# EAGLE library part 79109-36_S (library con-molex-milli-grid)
RECEPTACAL
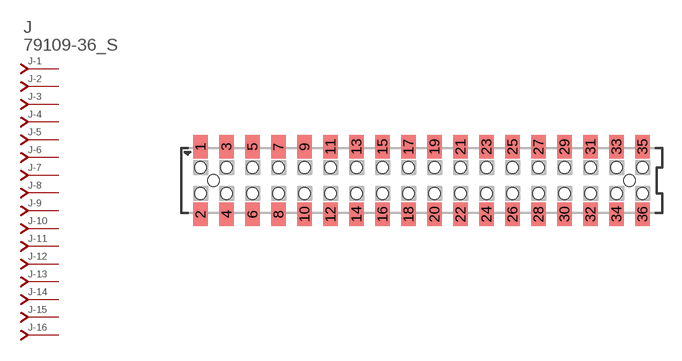
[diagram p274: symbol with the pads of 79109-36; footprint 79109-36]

Designator prefix J; gates -1=J-NV -2=J-N -3=J-N -4=J-N -5=J-N -6=J-N -7=J-N -8=J-N -9=J-N -10=J-N -11=J-N -12=J-N -13=J-N -14=J-N -15=J-N -16=J-N -17=J-N -18=J-N -19=J-N -20=J-N -21=J-N -22=J-N -23=J-N -24=J-N -25=J-N -26=J-N -27=J-N -28=J-N -29=J-N -30=J-N -31=J-N -32=J-N -33=J-N -34=J-N -35=J-N -36=J-N

## 79109-36_S  [79109-36]
1  -1:J  pas
2  -2:J  pas
3  -3:J  pas
4  -4:J  pas
5  -5:J  pas
6  -6:J  pas
7  -7:J  pas
8  -8:J  pas
9  -9:J  pas
10  -10:J  pas
11  -11:J  pas
12  -12:J  pas
13  -13:J  pas
14  -14:J  pas
15  -15:J  pas
16  -16:J  pas
17  -17:J  pas
18  -18:J  pas
19  -19:J  pas
20  -20:J  pas
21  -21:J  pas
22  -22:J  pas
23  -23:J  pas
24  -24:J  pas
25  -25:J  pas
26  -26:J  pas
27  -27:J  pas
28  -28:J  pas
29  -29:J  pas
30  -30:J  pas
31  -31:J  pas
32  -32:J  pas
33  -33:J  pas
34  -34:J  pas
35  -35:J  pas
36  -36:J  pas

## Footprint 79109-36 (pad centres in mm)
RECEPTACAL SMD Dual Row, Vertical, Pass-Thru
smd 1.12 x 1.83: 1 -17,2.6; 2 -17,-2.6; 3 -15,2.6; 4 -15,-2.6; 5 -13,2.6; 6 -13,-2.6; 7 -11,2.6; 8 -11,-2.6; 9 -9,2.6; 10 -9,-2.6; 11 -7,2.6; 12 -7,-2.6; 13 -5,2.6; 14 -5,-2.6; 15 -3,2.6; 16 -3,-2.6; 17 -1,2.6; 18 -1,-2.6; 19 1,2.6; 20 1,-2.6; 21 3,2.6; 22 3,-2.6; 23 5,2.6; 24 5,-2.6; 25 7,2.6; 26 7,-2.6; 27 9,2.6; 28 9,-2.6; 29 11,2.6; 30 11,-2.6; 31 13,2.6; 32 13,-2.6; 33 15,2.6; 34 15,-2.6; 35 17,2.6; 36 17,-2.6
hole 0.914 at -16,0
hole 0.914 at -17,1
hole 0.914 at -17,-1
hole 0.914 at -15,-1
hole 0.914 at -15,1
hole 0.914 at -13,-1
hole 0.914 at -13,1
hole 0.914 at 16,0
hole 0.914 at -11,1
hole 0.914 at -11,-1
hole 0.914 at -9,1
hole 0.914 at -9,-1
hole 0.914 at -7,1
hole 0.914 at -7,-1
hole 0.914 at -5,1
hole 0.914 at -5,-1
hole 0.914 at -3,-1
hole 0.914 at -3,1
hole 0.914 at -1,1
hole 0.914 at -1,-1
hole 0.914 at 1,1
hole 0.914 at 1,-1
hole 0.914 at 3,1
hole 0.914 at 3,-1
hole 0.914 at 5,-1
hole 0.914 at 5,1
hole 0.914 at 7,1
hole 0.914 at 9,1
hole 0.914 at 11,1
hole 0.914 at 7,-1
hole 0.914 at 9,-1
hole 0.914 at 11,-1
hole 0.914 at 13,-1
hole 0.914 at 15,-1
hole 0.914 at 17,-1
hole 0.914 at 13,1
hole 0.914 at 15,1
hole 0.914 at 17,1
